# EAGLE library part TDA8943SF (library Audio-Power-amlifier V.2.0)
6 W mono Bridge Tied Load (BTL) audio amplifier
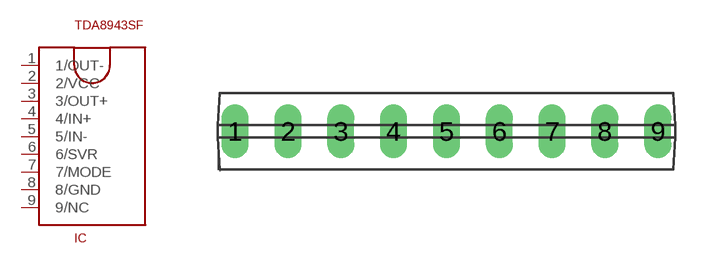
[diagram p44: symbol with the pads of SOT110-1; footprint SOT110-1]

Designator prefix IC

## TDA8943SF  [SOT110-1]
1  1/OUT-  out
2  2/VCC  pwr
3  3/OUT+  out
4  4/IN+  in
5  5/IN-  in
6  6/SVR
7  7/MODE
8  8/GND  pwr
9  9/NC  nc

## Footprint SOT110-1 (pad centres in mm)
SIL9MPF: plastic single in-line medium power package with fin; 9 leads
drill 0.8 long: 1 -10.16,0; 2 -7.62,0; 3 -5.08,0; 4 -2.54,0; 5 0,0; 6 2.54,0; 7 5.08,0; 8 7.62,0; 9 10.16,0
